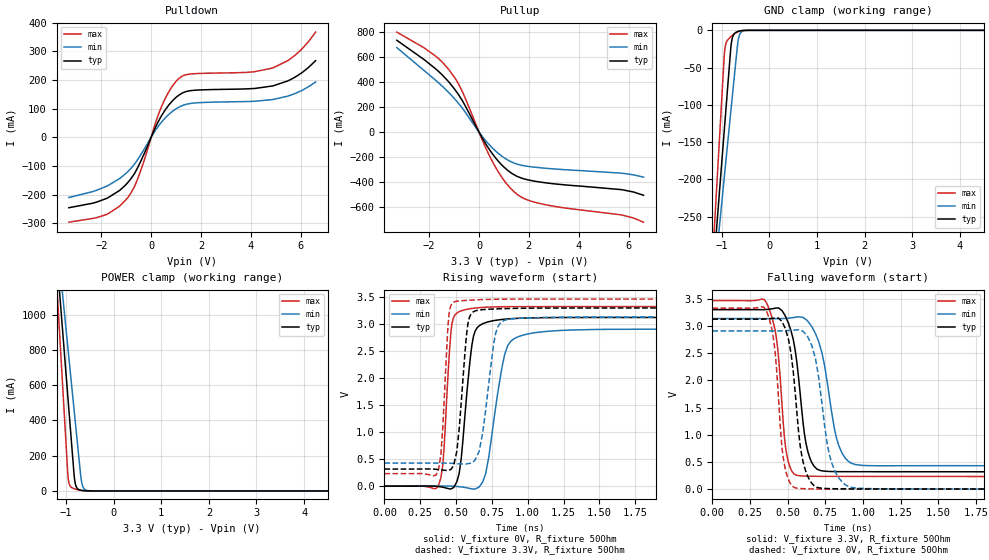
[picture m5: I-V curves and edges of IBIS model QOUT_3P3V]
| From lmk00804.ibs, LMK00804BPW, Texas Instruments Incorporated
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|   Model QOUT 3.3VCC
[Model]   QOUT_3P3V
Model_type   3-state
Polarity   Non-Inverting
Vmeas = 1.65
Vref = 3.3
Cref = 15pF
Rref = 50
|   typ   min   max
|   (fast PVT)   (slow PVT)   (nom PVT)
C_comp   0.315p   0.300p   0.317p
|C_comp (Hi state)   0.315p   0.300p   0.317p
|C_comp (Low state)   0.358p   0.325p   0.360p
[Voltage Range]   3.3   3.135   3.465
[Temperature Range]   45   125   -40
[Pullup Reference]   3.3   3.135   3.465
[Pulldown Reference]   0   0   0
[Power Clamp Reference]   3.3   3.135   3.465
[GND Clamp Reference]   0   0   0
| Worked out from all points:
|   slope of the pulldown table from 0 to 0.495 V, typ, clamps not added: 5.76 ohm
|   slope of the pullup table from 0 to 0.495 V, typ, clamps not added: 3.07 ohm
|   GND clamp passes 1 mA (typ) near -0.64 V on its own axis
|   POWER clamp passes 1 mA (typ) near -0.60 V on its own axis
|   falling waveform, V_fixture 3.3V, R_fixture 50Ohm: 20-80 % time 77.2ps typ, 103ps min, 58.8ps max; typ from 3.3 V to 0.318 V
|   rising waveform, V_fixture 0V, R_fixture 50Ohm: 20-80 % time 65.2ps typ, 99.8ps min, 43.5ps max; typ from 0 V to 3.12 V
|   rising waveform, V_fixture 3.3V, R_fixture 50Ohm: 20-80 % time 53.7ps typ, 75.9ps min, 38.5ps max; typ from 0.317 V to 3.3 V
|   falling waveform, V_fixture 0V, R_fixture 50Ohm: 20-80 % time 70.9ps typ, 93.1ps min, 55.9ps max; typ from 3.12 V to 0.001 V
[Pulldown]
|   Voltage   I(typ)   I(min)   I(max)
-3.3V     -245.4mA   -209.8mA   -295.9mA
-1.795V   -213.3mA   -170.8mA   -269.3mA
-924mV    -156.6mA   -118.7mA   -208.8mA
-528mV    -103.7mA   -76.1mA    -142.2mA
432.3mV   77.47mA    54.75mA    110.1mA
739.2mV   115.9mA    82.35mA    163.4mA
1.125V    148mA      105.7mA    206.3mA
1.68V     163.9mA    119.4mA    221.7mA
3.897V    169.4mA    125.1mA    227.2mA
4.887V    179.6mA    132.1mA    242.3mA
5.778V    210.1mA    152.9mA    286.3mA
6.6V      267.5mA    193mA      367.3mA
[GND Clamp]
|   Voltage   I(typ)   I(min)   I(max)
-3.3V     -2.075A    -1.751A    -2.656A
-1.231V   -364.5mA   -380.6mA   -346.8mA
-1.122V   -275mA     -309.3mA   -225.2mA
-1.112V   -266.8mA   -302.9mA   -214.2mA
-1.023V   -193.9mA   -244.8mA   -114.9mA
-933.9mV  -121.3mA   -187mA     -23.66mA
-805.2mV  -19.07mA   -104.2mA   -8.098mA
-765.6mV  -7.382mA   -78.94mA   -6.032mA
-676.5mV  -1.835mA   -22.61mA   -2.382mA
-617.1mV  -738uA     -4.371mA   -940.4uA
-488.4mV  -52.21uA   -146.8uA   -48.53uA
6.6V      0A         0A         0A
[Pullup]
|   Voltage   I(typ)   I(min)   I(max)
-3.3V     731.9mA    673.5mA    796.9mA
-1.716V   500mA      409mA      602mA
-1.181V   392.2mA    308.4mA    490.4mA
-676.5mV  253.1mA    192.6mA    325.8mA
125.4mV   -45.29mA   -33.15mA   -60.57mA
570.9mV   -182mA     -133.2mA   -246.9mA
1.086V    -294.1mA   -214.5mA   -406.2mA
1.541V    -353.7mA   -256.1mA   -497.2mA
1.947V    -379.9mA   -272.6mA   -540.9mA
2.511V    -399.8mA   -285.2mA   -572.2mA
5.709V    -458.4mA   -327.2mA   -659.8mA
6.6V      -503.3mA   -358.8mA   -718mA
[POWER Clamp]
|   Voltage   I(typ)   I(min)   I(max)
-3.3V     8.665A     7.319A     11.12A
-1.31V    1.725A     1.766A     1.709A
-1.053V   843mA      1.061A     510mA
-953.7mV  506.1mA    792mA      70.2mA
-924mV    405.3mA    711.4mA    32.29mA
-834.9mV  103.8mA    470.2mA    13.02mA
-815.1mV  55.25mA    416.7mA    11.19mA
-785.4mV  23.71mA    336.7mA    8.755mA
-676.5mV  3.313mA    55.79mA    2.559mA
-636.9mV  1.849mA    18.74mA    1.374mA
-557.7mV  449.8uA    2.365mA    292.6uA
6.6V      0A         0A         0A
[Ramp]
R_load = 50
|   typ   min   max
dV/dt_r   1.87446/6.52328e-11   1.74494/9.98179e-11   1.99586/4.34514e-11
dV/dt_f   1.78949/7.72046e-11   1.62421/1.03258e-10   1.93985/5.87796e-11
[Falling Waveform]
V_fixture = 3.3V
V_fixture_min = 3.135V
V_fixture_max = 3.465V
R_fixture = 50Ohm
C_fixture = 0F
|   Time   V(typ)   V(min)   V(max)
0s        3.3V       3.135V     3.465V
361.2ps   3.303V     3.134V     3.417V
426.2ps   3.328V     3.133V     2.76V
493.5ps   3.125V     3.141V     639.8mV
560.5ps   2.341V     3.164V     255.2mV
611ps     1.021V     3.139V     240.4mV
659.4ps   494mV      2.991V     237mV
839.5ps   322.2mV    799.8mV    235.3mV
947.3ps   321.5mV    454mV      235.1mV
3.9ns     317.5mV    428mV      231.9mV
[Rising Waveform]
V_fixture = 0V
V_fixture_min = 0V
V_fixture_max = 0V
R_fixture = 50Ohm
C_fixture = 0F
|   Time   V(typ)   V(min)   V(max)
0s        476.5pV    13.15nV    450.3pV
378.5ps   -8.06mV    1.638mV    23.78mV
407.3ps   -19.46mV   1.763mV    388.8mV
470.2ps   -43.43mV   616uV      2.992V
542.7ps   706.8mV    -15.56mV   3.253V
634.1ps   2.878V     -50.33mV   3.299V
705.9ps   3.028V     222.9mV    3.313V
839.5ps   3.092V     2.44V      3.323V
947.3ps   3.11V      2.78V      3.325V
3.9ns     3.124V     2.908V     3.326V
[Rising Waveform]
V_fixture = 3.3V
V_fixture_min = 3.135V
V_fixture_max = 3.465V
R_fixture = 50Ohm
C_fixture = 0F
|   Time   V(typ)   V(min)   V(max)
0s        316.9mV    426.7mV    231.6mV
378.5ps   306.5mV    427.8mV    318mV
407.3ps   297.7mV    427.4mV    1.083V
450ps     297.4mV    425.5mV    3.168V
493.5ps   504.1mV    418.1mV    3.417V
583.1ps   3.014V     417.2mV    3.443V
634.1ps   3.246V     495.3mV    3.45V
776.5ps   3.282V     2.833V     3.461V
839.5ps   3.288V     3.073V     3.462V
3.9ns     3.3V       3.134V     3.465V
[Falling Waveform]
|Gnd
V_fixture = 0V
V_fixture_min = 0V
V_fixture_max = 0V
R_fixture = 50Ohm
C_fixture = 0F
|   Time   V(typ)   V(min)   V(max)
0s        3.125V     2.909V     3.327V
361.2ps   3.128V     2.909V     3.263V
417.3ps   3.146V     2.908V     2.506V
470.2ps   3.035V     2.911V     587.7mV
542.7ps   1.993V     2.924V     31.81mV
583.1ps   798.6mV    2.918V     12.63mV
647.9ps   157.2mV    2.714V     5.712mV
791.4ps   8.838mV    491.6mV    3.33mV
919.6ps   4.98mV     35mV       3.044mV
3.9ns     536.7uV    965.6uV    295.7uV
